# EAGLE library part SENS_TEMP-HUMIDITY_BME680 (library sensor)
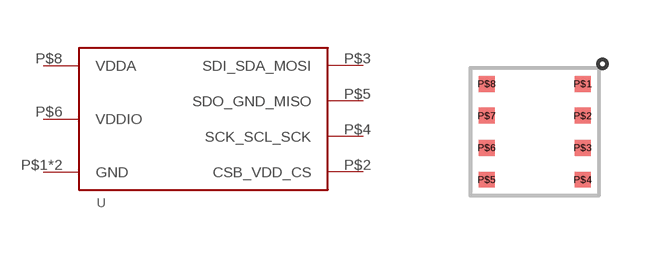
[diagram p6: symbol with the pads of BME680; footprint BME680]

Designator prefix U

## SENS_TEMP-HUMIDITY_BME680  [BME680]
P$1  GND
P$2  CSB_VDD_CS
P$3  SDI_SDA_MOSI
P$4  SCK_SCL_SCK
P$5  SDO_GND_MISO
P$6  VDDIO
P$7  GND
P$8  VDDA

## Footprint BME680 (pad centres in mm)
smd 0.4 x 0.4: P$1 1.2,1.2; P$2 1.2,0.4; P$3 1.2,-0.4; P$4 1.2,-1.2; P$5 -1.2,-1.2; P$6 -1.2,-0.4; P$7 -1.2,0.4; P$8 -1.2,1.2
